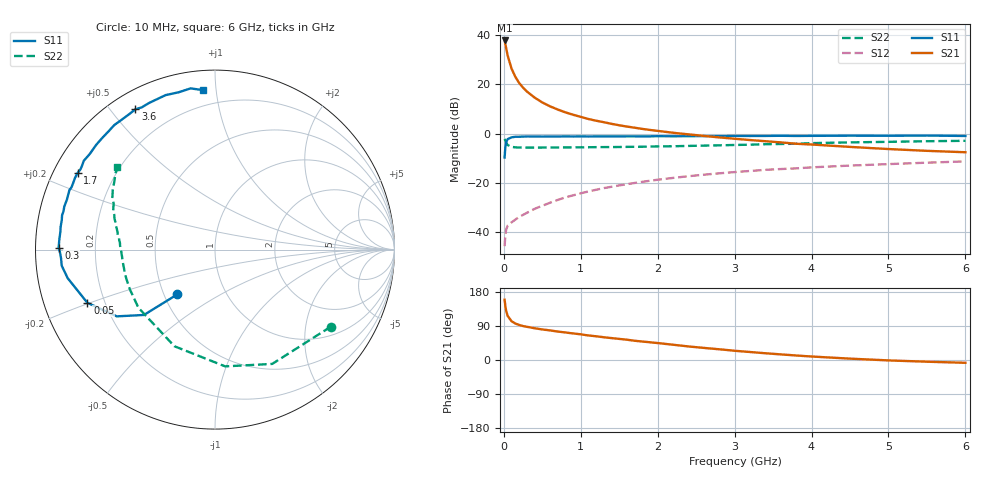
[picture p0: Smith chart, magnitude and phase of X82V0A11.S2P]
! SIEMENS Small Signal Semiconductors
! BFP136W
! Si NPN RF Bipolar Junction Transistor in SOT343
! VCE = 2 V  IC = 110 mA
! Common Emitter S-Parameters:  September  1994
# GHz  S  MA  R  50
!  f  S11  S21  S12  S22
! GHz  MAG  ANG  MAG  ANG  MAG  ANG  MAG  ANG
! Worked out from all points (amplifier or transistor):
!   40 points, 10 MHz to 6 GHz, reference 50 ohm
!   highest |S21| = 37.7 dB at 10 MHz (marker M1)
!   |S21| within 3 dB of that: start of sweep to 29.5 MHz
!   unconditionally stable (mu >= 1): 452.7 MHz to 2.91 GHz
!   at 200 MHz: K = 0.74, MSG = 27.1 dB, |S12| = -33.8 dB
!   at 1.5 GHz: K = 1.11, MAG = 10.2 dB, |S12| = -21.0 dB
!   at 6 GHz: K = 0.99, MSG = 1.9 dB, |S12| = -11.3 dB
!   S11 on the Smith chart (normalised r, x): 10 MHz: 0.59, -0.33; 50 MHz: 0.13, -0.20; 300 MHz: 0.07, +0.01; 1.7 GHz: 0.07, +0.26; 3.6 GHz: 0.07, +0.58; 6 GHz: 0.11, +0.92
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0.01  0.3264 -130.1  76.94 159.0  0.0052 67.1  0.7753 -33.6
0.02  0.538 -137.4  65.06 141.8  0.0088 55.5  0.7122 -63.4
0.03  0.6617 -145.8  53.96 130.0  0.0112 47.3  0.6531 -85.0
0.05  0.7705 -157.4  37.9 116.2  0.0136 38.5  0.584 -112.8
0.1  0.8359 -169.0  20.69 102.3  0.0158 36.6  0.5357 -142.8
0.15  0.8586 -174.0  14.04 96.2  0.018 41.2  0.5235 -154.8
0.2  0.8592 -176.8  10.53 92.4  0.0204 44.1  0.52 -161.3
0.25  0.8648 -179.3  8.489 89.6  0.0224 47.7  0.5195 -165.3
0.3  0.8715 179.3  7.099 87.6  0.0247 50.7  0.5177 -168.1
0.4  0.869 175.9  5.344 83.8  0.0297 54.9  0.5182 -171.8
0.5  0.867 173.4  4.259 80.6  0.0343 57.8  0.5189 -174.3
0.6  0.8694 171.7  3.556 78.1  0.0394 59.9  0.5195 -176.0
0.8  0.8731 167.4  2.684 72.7  0.0507 62.3  0.5223 -178.6
1.1  0.8708 161.4  1.967 64.7  0.0668 62.8  0.5265 178.6
1.4  0.8717 156.5  1.57 57.8  0.0832 62.0  0.5304 176.2
1.7  0.8764 150.8  1.31 50.8  0.0994 60.2  0.5377 173.7
2.2  0.8779 142.6  1.035 40.3  0.1258 56.0  0.5515 169.9
3.2  0.8911 125.6  0.737 21.1  0.1739 46.0  0.5935 161.0
3.6  0.8985 119.6  0.661 14.8  0.1903 42.0  0.6131 157.5
4.5  0.9037 107.7  0.535 3.6  0.2236 33.3  0.6608 149.5
5.5  0.9084 98.6  0.445 -4.5  0.2562 25.3  0.6973 142.8
6  0.8911 94.3  0.417 -7.4  0.2721 20.8  0.711 139.9
